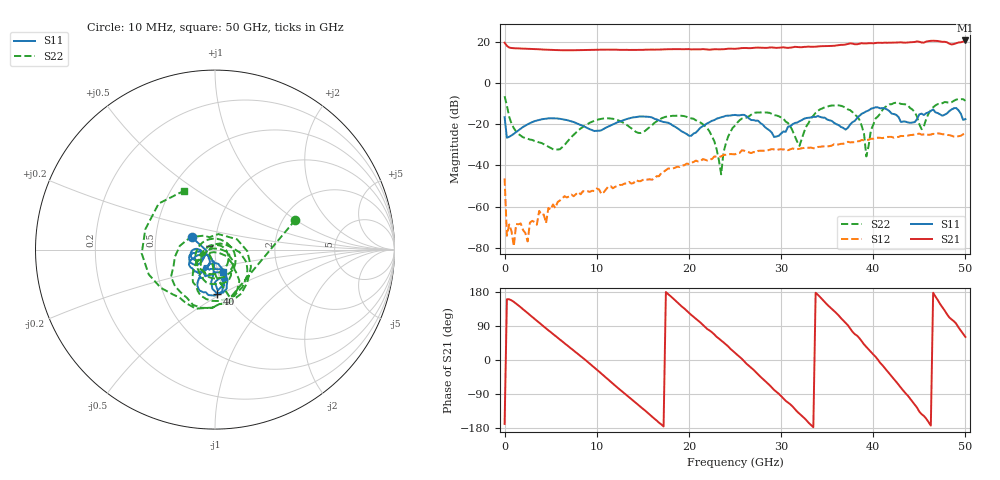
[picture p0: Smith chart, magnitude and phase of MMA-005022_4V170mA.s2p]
!Agilent Technologies,E8364B,MY43030235,A.06.04.32
!Agilent E8364B: A.06.04.32
!Date: Monday, February 27, 2012 16:19:05
!Correction: S11(Full 2 Port(1,2)) S21(Full 2 Port(1,2)) S12(Full 2 Port(1,2)) S22(Full 2 Port(1,2))
!S2P File: Measurements: S11, S21, S12, S22:
# Hz S  dB  R 50
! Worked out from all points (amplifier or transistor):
!   201 points, 10 MHz to 50 GHz, reference 50 ohm
!   highest |S21| = 20.6 dB at 50 GHz (marker M1)
!   |S21| within 3 dB of that: 33.81 GHz to end of sweep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
!   unconditionally stable (mu >= 1): start of sweep to 49.97 GHz
!   at 8.258 GHz: K = 39.38, MAG = 16.0 dB, |S12| = -54.0 dB
!   at 25 GHz: K = 3.90, MAG = 16.8 dB, |S12| = -34.6 dB
!   at 50 GHz: K = 0.99, MSG = 22.4 dB, |S12| = -24.1 dB
!   S11 on the Smith chart (normalised r, x): 10 MHz: 0.76, +0.11; 40 GHz: 0.91, -0.48; 50 GHz: 1.06, -0.27
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1e7  -16.61 151.9  19.54 -168.8  -46.33 -5.9  -6.41 20.4
2.5995e8  -26.58 -172.2  18.02 160.4  -74.11 -103.5  -11.01 -72.5
3.75925e9  -17.91 -153.8  16.36 98.3  -62.06 -164.1  -28.83 -158.0
8.5083e9  -20.89 179.2  15.97 5.3  -52.48 72.0  -21.30 -29.6
1.275745e10  -18.30 -138.6  16.08 -82.7  -49.44 -15.1  -18.97 -164.8
1.675665e10  -18.16 -171.6  16.22 -165.3  -45.24 -104.2  -17.94 -25.7
1.85063e10  -21.25 -173.3  16.49 157.6  -41.09 -150.0  -15.93 -78.5
2.15057e10  -20.98 -111.6  16.45 93.0  -36.95 147.5  -19.96 -142.2
2.5005e10  -15.49 -136.4  16.59 19.2  -34.61 80.5  -20.67 -25.6
2.70046e10  -18.01 -153.6  17.05 -25.6  -33.51 45.2  -14.59 -65.6
2.925415e10  -26.22 -139.4  17.16 -79.1  -32.26 -9.7  -15.59 -114.5
3.15037e10  -19.39 -93.7  17.56 -129.5  -31.99 -62.4  -25.85 173.7
3.35033e10  -16.41 -106.0  17.57 -177.4  -31.66 -113.4  -15.87 -14.7
3.575285e10  -19.33 -122.9  18.06 129.3  -29.72 -173.1  -10.96 -80.4
3.75025e10  -20.12 -72.8  19.22 83.0  -28.82 136.7  -13.17 -124.0
4.0002e10  -12.13 -87.2  19.26 14.7  -27.04 73.6  -20.30 -35.7
4.175165e10  -13.60 -117.9  19.54 -36.3  -26.15 25.2  -10.36 -77.7
4.30014e10  -18.92 -116.7  19.73 -73.4  -25.70 -9.7  -10.16 -120.5
4.425115e10  -19.18 -84.7  19.83 -109.4  -25.19 -46.4  -12.89 -169.9
4.65007e10  -12.84 -86.2  20.50 177.4  -24.66 -127.2  -11.80 -45.7
4.80004e10  -14.76 -67.3  19.74 121.0  -25.22 170.1  -9.39 -118.5
5e10  -17.53 -70.9  20.64 60.9  -24.14 108.6  -8.62 118.1
